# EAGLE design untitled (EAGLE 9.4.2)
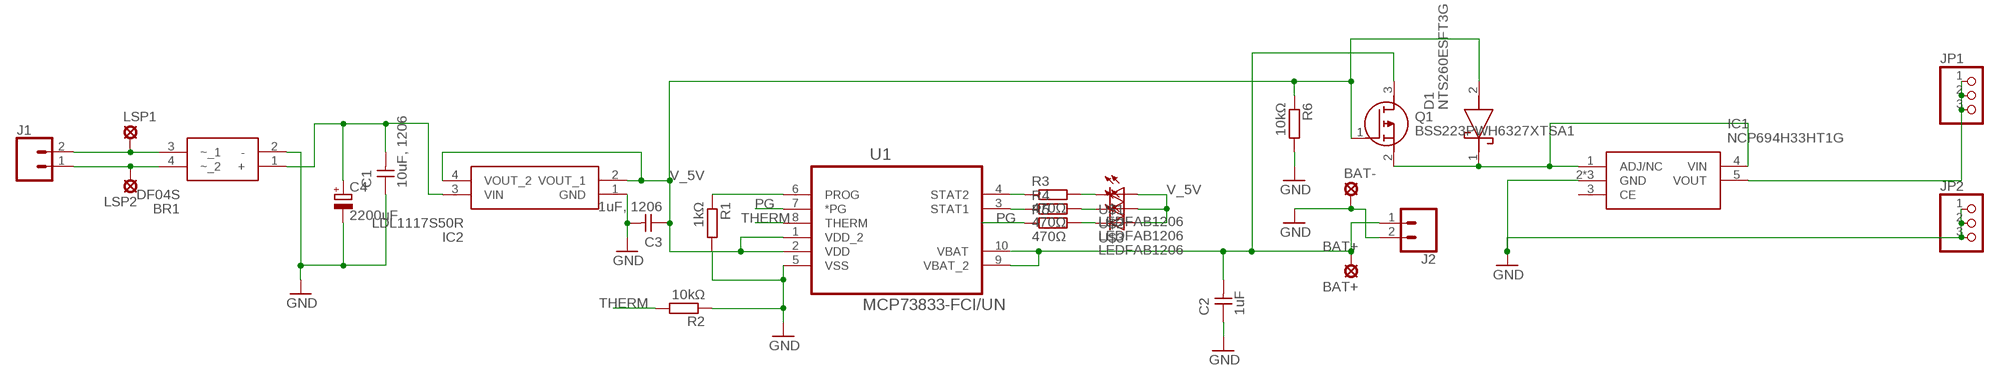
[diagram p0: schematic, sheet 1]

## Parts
BAT+  LSP10  [LSP10]
BAT-  LSP10  [LSP10]
BR1  DF04S  [SOP510P985X293-4N]
C1  10uF, 1206  CAP-UNPOLARIZEDFAB  [C1206FAB]
C2  1uF  CAP-UNPOLARIZEDFAB  [C1206FAB]
C3  1uF, 1206  CAP-UNPOLARIZEDFAB  [C1206FAB]
C4  2200uF  CPOL-EUE5-10.5  [E5-10,5]
D1  NTS260ESFT3G  [SODFL3616X98N]
IC1  NCP694H33HT1G  [ON_SOT-89]
IC2  LDL1117S50R  [SOT230P700X180-4N]
J1  CONN_025MM  [SCREWTERMINAL-5MM-2]
J2  CONN_025MM  [SCREWTERMINAL-5MM-2]
JP1  PINHD-1X3  [1X03]
JP2  PINHD-1X3  [1X03]
LSP1  LSP10  [LSP10]
LSP2  LSP10  [LSP10]
Q1  BSS223PWH6327XTSA1  [SOT65P210X100-3N]
R1  1kΩ  R-EU_R0603  [R0603]
R2  10kΩ  R-EU_R0603  [R0603]
R3  470Ω  R-EU_R0603  [R0603]
R4  470Ω  R-EU_R0603  [R0603]
R5  470Ω  R-EU_R0603  [R0603]
R6  10kΩ  R-EU_R0603  [R0603]
U1  MCP73833-FCI/UN  [SOP50P490X110-10N]
U$1  LEDFAB1206  [LED1206FAB]
U$2  LEDFAB1206  [LED1206FAB]
U$3  LEDFAB1206  [LED1206FAB]

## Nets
BAT+: BAT+.MP C2.2 J2.1 Q1.3(D) U1.9(VBAT_2) U1.10(VBAT)
GND: BAT-.MP BR1.2(-) C1.1 C2.1 C3.2 C4.- IC1.2(GND) IC1.6(GND) IC1.7(GND) IC2.1(GND) J2.2 JP2.1 JP2.2 JP2.3 R1.2 R2.1 R6.2 U1.5(VSS)
N$1: IC1.5(VOUT) JP1.1 JP1.2 JP1.3
N$2: BR1.3(~_1) J1.2 LSP1.MP
N$3: BR1.1(+) C1.2 C4.+ IC2.3(VIN)
N$4: BR1.4(~_2) J1.1 LSP2.MP
N$5: R1.1 U1.6(PROG)
N$6: R3.2 U$1.2(C)
N$7: R3.1 U1.4(STAT2)
N$8: R4.1 U1.3(STAT1)
N$9: R5.2 U$3.2(C)
N$10: R4.2 U$2.2(C)
N$11: D1.1(K) IC1.1(ADJ/NC) IC1.4(VIN) Q1.2(S)
PG: R5.1 U1.7(*PG)
THERM: R2.2 U1.8(THERM)
V_5V: C3.1 D1.2(A) IC2.2(VOUT_1) IC2.4(VOUT_2) Q1.1(G) R6.1 U1.1(VDD_2) U1.2(VDD) U$1.1(A) U$2.1(A) U$3.1(A)
Unconnected: IC1.3(CE)

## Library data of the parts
BAT+ BAT- LSP1 LSP2 = solpad:LSP10: SOLDER PAD
BR1 = SamacSys_Parts:DF04S: ON Semiconductor DF04S, Bridge Rectifier, 1.5A 400V, 4-Pin SDIP Source: Datasheet; DESCRIPTION: ON Semiconductor DF04S, Bridge Rectifier, 1.5A 400V, 4-Pin SDIP; HEIGHT: 2.93mm; MANUFACTURER_NAME: ON Semiconductor; MANUFACTURER_PART_NUMBER: DF04S; MOUSER_PART_NUMBER: 512-DF04S
C1-C3 = fab:CAP-UNPOLARIZED
C4 = rcl:CPOL-EU: POLARIZED CAPACITOR, European symbol; SPICEPREFIX: C
D1 = SamacSys_Parts:NTS260ESFT3G: Schottky Diodes & Rectifiers 2A 60V LOW LEAKAGE TRENC; DESCRIPTION: Schottky Diodes & Rectifiers 2A 60V LOW LEAKAGE TRENC; HEIGHT: 0.98mm; MANUFACTURER_NAME: ON Semiconductor; MANUFACTURER_PART_NUMBER: NTS260ESFT3G; MOUSER_PART_NUMBER: 863-NTS260ESFT3G; MOUSER_PRICE-STOCK: https://www.mouser.com/Search/Refine.aspx?Keyword=863-NTS260ESFT3G
IC1 = SamacSys_Parts:NCP694H33HT1G: ON Semiconductor NCP694H33HT1G, LDO Voltage Regulator, 1A, 3.3 V, 1.4 6 Vin, 5-Pin SOT-89 Source: Datasheet; DESCRIPTION: ON Semiconductor NCP694H33HT1G, LDO Voltage Regulator, 1A, 3.3 V, 1.4 6 Vin, 5-Pin SOT-89; HEIGHT: mm; MANUFACTURER_NAME: ON Semiconductor; MANUFACTURER_PART_NUMBER: NCP694H33HT1G; MOUSER_PART_NUMBER: 863-NCP694H33HT1G; MOUSER_PRICE-STOCK: https://www.mouser.com/Search/Refine.aspx?Keyword=863-NCP694H33HT1G
IC2 = SamacSys_Parts:LDL1117S50R: STMICROELECTRONICS - LDL1117S50R - LDO, FIXED, 5V, 1.2A, SOT-223-3 Source: Datasheet; DESCRIPTION: STMICROELECTRONICS - LDL1117S50R - LDO, FIXED, 5V, 1.2A, SOT-223-3; HEIGHT: 1.8mm; MANUFACTURER_NAME: STMicroelectronics; MANUFACTURER_PART_NUMBER: LDL1117S50R; MOUSER_PART_NUMBER: 511-LDL1117S50R; MOUSER_PRICE-STOCK: https://www.mouser.com/Search/Refine.aspx?Keyword=511-LDL1117S50R
J1 J2 = SparkFun-Connectors:CONN_02: Multi connection point. Often used as Generic Header-pin footprint for 0.1 inch spaced/style header connections; SF_SKU: PRT-08432
JP1 JP2 = pinhead+:PINHD-1X3: PIN HEADER
Q1 = SamacSys_Parts:BSS223PWH6327XTSA1: Infineon BSS223PWH6327XTSA1 P-channel MOSFET Transistor, 0.31 A, -20 V, 3-Pin SOT-323 Source: Datasheet; DESCRIPTION: Infineon BSS223PWH6327XTSA1 P-channel MOSFET Transistor, 0.31 A, -20 V, 3-Pin SOT-323; HEIGHT: 1mm; MANUFACTURER_NAME: Infineon; MANUFACTURER_PART_NUMBER: BSS223PWH6327XTSA1; MOUSER_PART_NUMBER: 726-BSS223PWH6327XTS; MOUSER_PRICE-STOCK: https://www.mouser.com/Search/Refine.aspx?Keyword=726-BSS223PWH6327XTS
R1-R6 = rcl:R-EU_: RESISTOR, European symbol; SPICEPREFIX: R
U1 = Microchip-MCP73833-FCI_UN:MCP73833-FCI/UN: LI-ION/LI-POLY CONTROLLERS; MPN: MCP73833-FCI/UN; OC_FARNELL: 1605576; OC_NEWARK: 88K5666; PACKAGE: MSOP10; SUPPLIER: Microchip
U$1-U$3 = fab:LED: LED

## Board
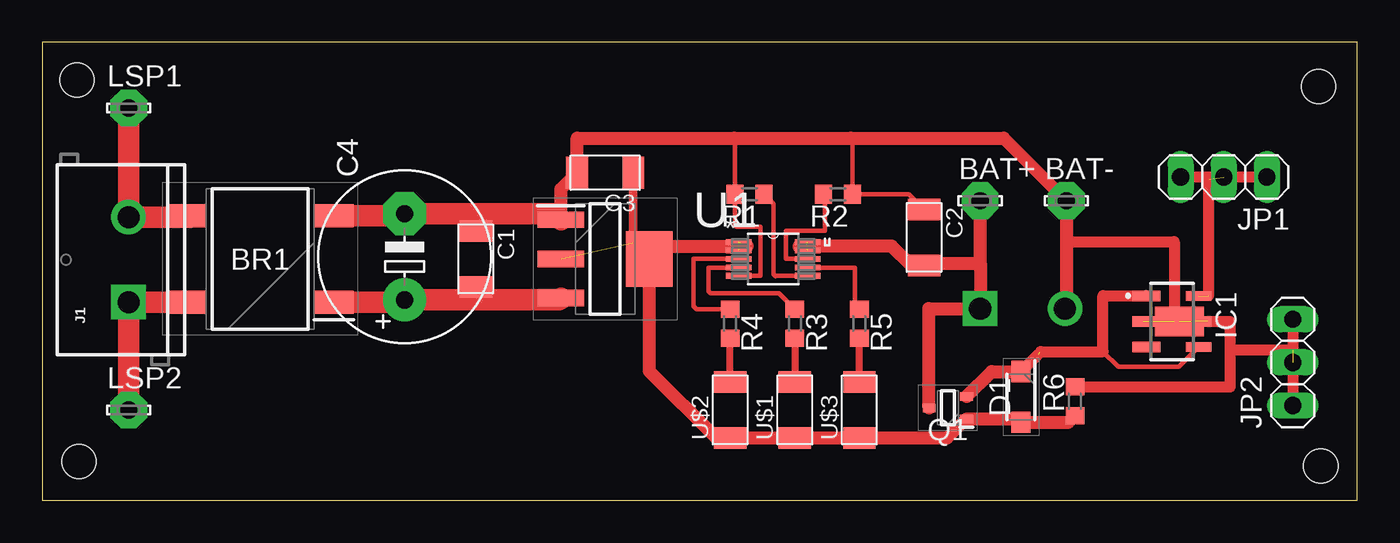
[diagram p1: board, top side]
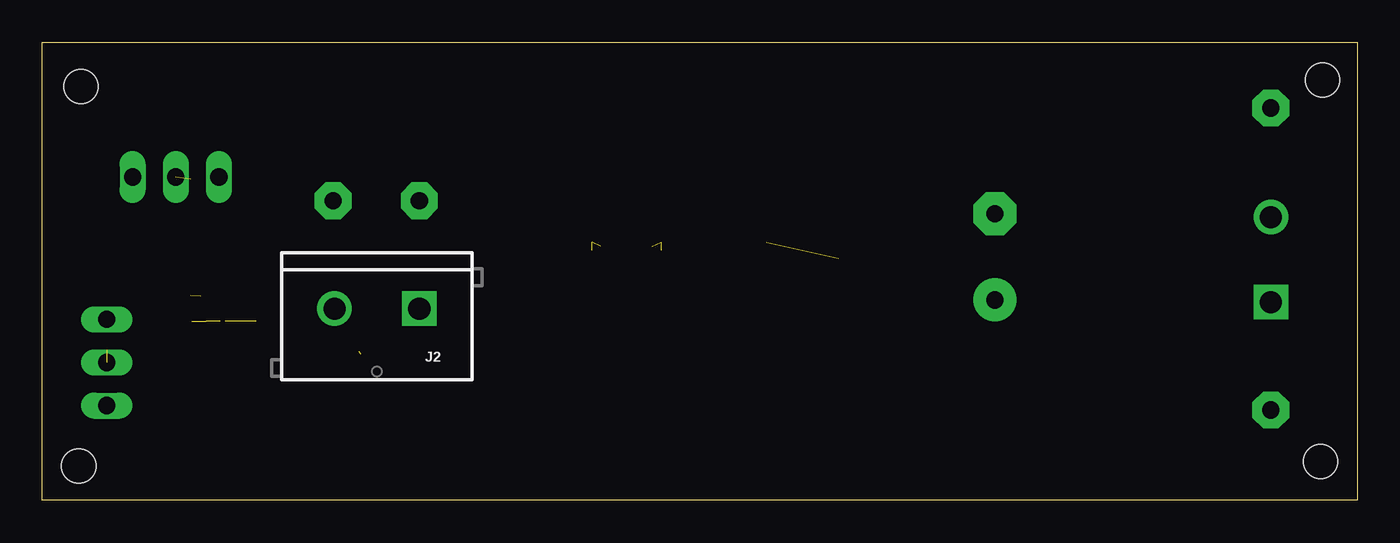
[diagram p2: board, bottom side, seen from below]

Size 77.45 x 26.98 mm. Coordinates in mm from the lower left corner, seen from the top.
Outline: 0,0 77.45,0 77.45,26.98 0,26.98 0,0
Copper layers (1*16): Top 0.035mm / dielectric 1.5mm / Bottom 0.035mm
Design rules "default": minimum track width 6mil, minimum drill 0.35mm, track to track 6mil, track to pad 6mil, pad to pad 6mil, via to via 6mil, smd to smd 6mil, copper to edge 40mil, drill to drill 6mil, minimum pad ring 10mil, minimum via ring 8mil, stop-mask expansion 4mil, vias tented up to drill 0mil, thermal gap 10mil
Holes 2 mm at 2.03,24.77 2.16,2.29 75.31,2.03 75.18,24.38

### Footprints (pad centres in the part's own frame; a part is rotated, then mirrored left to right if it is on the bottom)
LSP10 = drill 1.016 pad 2.159 octagon: MP 0,0
SOP510P985X293-4N = smd 2.325 x 1.35: 1 -4.338,2.55; 2 -4.338,-2.55; 3 4.338,-2.55; 4 4.338,2.55
C1206FAB = smd 1.27 x 1.905: 1 -1.651,0; 2 1.651,0
E5-10,5 = drill 1.016 pad 2.54: + -2.54,0 | drill 1.016 pad 2.54 octagon: - 2.54,0
SODFL3616X98N = smd 1.24 x 1.12: 1 -1.5,0; 2 1.5,0
ON_SOT-89 = smd 0.62 x 1.65: 1 -1.5,-1.5; 3 1.5,-1.5 | smd 0.62 x 1.3: 2 0,-1.675 | smd 0.57 x 1.5: 4 1.5,1.575; 5 -1.5,1.575 | smd 1.75 x 2.9: 6 0,0.425 | smd 0.57 x 0.45: 7 0,2.1
SOT230P700X180-4N = smd 2.75 x 0.95: 1 -2.6,2.3; 2 -2.6,0; 3 -2.6,-2.3 | smd 2.75 x 3.25: 4 2.6,0
SCREWTERMINAL-5MM-2 = drill 1.3 pad 2.032 square: 1 0,0 | drill 1.3 pad 2.032: 2 5,0
1X03 = drill 1.016 long: 1 -2.54,0; 2 0,0; 3 2.54,0
SOT65P210X100-3N = smd 0.75 x 0.5: 1 -1.1,0.65; 2 -1.1,-0.65; 3 1.1,0
R0603 = smd 1 x 1.1: 1 -0.85,0; 2 0.85,0
SOP50P490X110-10N = smd 1.524 x 0.33: 1 -2.032,0.991; 2 -2.032,0.508; 3 -2.032,0; 4 -2.032,-0.508; 5 -2.032,-0.991; 6 2.032,-0.991; 7 2.032,-0.508; 8 2.032,0; 9 2.032,0.508; 10 2.032,0.991
LED1206FAB = smd 1.27 x 1.905: 1 -1.651,0; 2 1.651,0

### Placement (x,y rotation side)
BAT+  55.24,17.65 0 top
BAT-  60.32,17.65 0 top
BR1  12.83,14.22 180 top
C1  25.53,14.22 270 top
C2  51.94,15.49 270 top
C3  33.15,19.3 180 top
C4  21.34,14.35 90 top
D1  57.66,6.1 270 top
IC1  66.55,10.54 270 top
IC2  33.15,14.22 0 top
J1  5.08,11.68 90 top
J2  55.24,11.3 180 bottom
JP1  69.6,19.05 180 top
JP2  73.66,8.13 90 top
LSP1  5.08,23.11 0 top
LSP2  5.08,5.33 0 top
Q1  53.34,5.46 180 top
R1  41.66,18.03 180 top
R2  46.86,18.03 180 top
R3  44.32,10.41 270 top
R4  40.51,10.41 270 top
R5  48.13,10.41 270 top
R6  60.83,5.84 90 top
U1  43.05,14.22 0 top
U$1  44.32,5.33 90 top
U$2  40.51,5.33 90 top
U$3  48.13,5.33 90 top

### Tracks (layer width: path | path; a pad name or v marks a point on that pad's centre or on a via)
BAT+  (2 unrouted)
  Top 0.762: 44.58,14.92 44.58,14.99 50.04,14.99 51.18,13.84 C2.2 52.07,13.97 55.24,13.97 | 55.24,13.97 J2.1 52.2,11.3 52.24,11.26 Q1.3 | 55.24,13.97 BAT+.MP
GND  (4 unrouted)
  Top 0.254: U1.5 42.29,13.23 42.29,16.13 40.89,16.13 40.81,16.22 R1.2 40.81,21.3 40.77,21.34 | 47.63,21.34 47.71,21.25 R2.1 51.05,18.03 C2.1
  Top 0.635: R6.2 69.98,6.69 69.98,8.89 | 69.98,8.89 69.98,10.54 67.82,10.54 | 60.45,15.24 66.68,15.24 66.68,10.54 | JP2.3 73.66,8.89 | 73.66,8.89 JP2.1 | 69.98,8.89 73.66,8.89
  Top 0.762: IC2.1 30.55,18.35 C3.2 31.5,21.34 40.77,21.34 47.63,21.34 56.64,21.34 BAT-.MP 60.32,15.11 | 60.32,15.11 60.32,11.38 | 60.32,15.11 60.45,15.24 | 66.68,10.54 IC1.6
  Top 1.27: BR1.2 21.22,16.77 C4.- 25.53,16.89 | 25.53,16.89 30.18,16.89 IC2.1 | 25.53,16.89 C1.1 | 60.32,11.38 J2.2
N$1  (2 unrouted)
  Top 0.635: JP1.1 68.58,19.05 | 68.58,19.05 JP1.3 | 68.58,19.05 68.71,18.92 68.71,12.06
N$2
  Top 1.27: BR1.3 8.62,16.77 8.71,16.68 J1.2 LSP1.MP
N$3
  Top 1.27: BR1.1 21.2,11.67 C4.+ 25.53,11.81 | 25.53,11.81 30.43,11.81 IC2.3 | 25.53,11.81 C1.2
N$4
  Top 1.27: LSP2.MP J1.1 BR1.4
N$5
  Top 0.254: U1.6 43.2,13.23 43.18,13.21 43.08,13.31 43.08,17.46 R1.1
N$6
  Top 0.406: R3.2 U$1.2
N$7
  Top 0.254: R3.1 43.4,12.19 39.37,12.19 39.24,12.32 39.24,13.72 U1.4
N$8
  Top 0.254: R4.1 38.52,11.26 38.35,11.43 38.35,14.22 U1.3
N$9
  Top 0.406: U$3.2 R5.2
N$10
  Top 0.406: U$2.2 R4.2
N$11  (1 unrouted)
  Top 0.254: IC1.4 66.96,7.87 63.37,7.87 62.48,8.76
  Top 0.635: D1.1 58.67,8.61 | 58.8,8.76 62.48,8.76 62.48,12.06 65.02,12.06 IC1.1
  Top 0.762: Q1.2 55.93,7.6 D1.1
PG
  Top 0.254: R5.1 47.88,11.52 47.88,13.72 U1.7
THERM
  Top 0.254: U1.8 43.82,14.22 43.82,15.88 46.1,15.88 46.1,17.95 R2.2
V_5V  (3 unrouted)
  Top 0.406: U$3.1 U$1.1 U$2.1 39.68,3.68
  Top 0.508: C3.1 34.8,15.17 IC2.4
  Top 0.762: 41.53,14.99 36.51,14.99 IC2.4 35.75,7.62 39.68,3.68 | U$2.1 U$3.1 53.31,3.68 Q1.1 57.44,4.81 D1.2 60.44,4.6 R6.1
